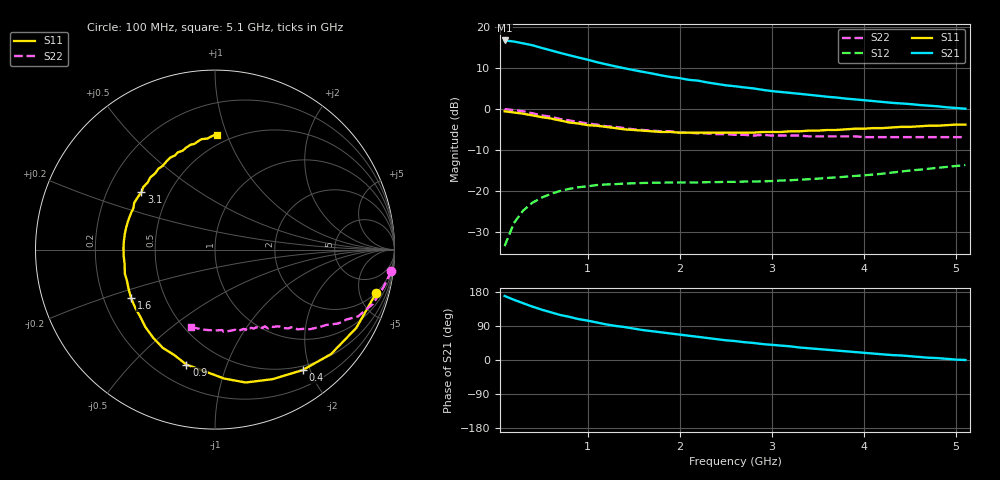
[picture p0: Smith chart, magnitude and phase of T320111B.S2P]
!AT-32011
!S PARAMETERSat Vce=1 V  Ic=2mA.  LAST UPDATED 01-05-95
# ghz s ma r 50
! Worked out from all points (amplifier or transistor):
!   51 points, 100 MHz to 5.1 GHz, reference 50 ohm
!   highest |S21| = 16.7 dB at 100 MHz (marker M1)
!   |S21| within 3 dB of that: start of sweep to 696.7 MHz
!   unconditionally stable (mu >= 1): 2.379 GHz to end of sweep
!   at 900 MHz: K = 0.39, MSG = 15.8 dB, |S12| = -19.2 dB
!   at 2.6 GHz: K = 1.08, MAG = 10.0 dB, |S12| = -17.9 dB
!   at 5.1 GHz: K = 1.06, MAG = 5.4 dB, |S12| = -13.8 dB
!   S11 on the Smith chart (normalised r, x): 100 MHz: 1.98, -7.05; 400 MHz: 0.44, -1.88; 900 MHz: 0.32, -0.73; 1.6 GHz: 0.32, -0.24; 3.1 GHz: 0.35, +0.31; 5.1 GHz: 0.43, +0.92
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0.1  0.93 -15.0  6.81 169.0  0.021 82.0  0.99 -7.0
0.2  0.9 -29.0  6.61 159.0  0.04 74.0  0.96 -13.0
0.3  0.87 -42.0  6.28 150.0  0.057 66.0  0.93 -19.0
0.4  0.83 -54.0  5.96 141.0  0.071 60.0  0.88 -25.0
0.5  0.79 -66.0  5.53 133.0  0.082 54.0  0.83 -28.0
0.6  0.76 -77.0  5.16 126.0  0.091 49.0  0.8 -31.0
0.7  0.72 -86.0  4.81 119.0  0.099 45.0  0.75 -34.0
0.9  0.66 -104.0  4.22 108.0  0.11 38.0  0.69 -40.0
1  0.63 -111.0  3.97 104.0  0.113 36.0  0.66 -42.0
1.2  0.6 -125.0  3.49 94.0  0.119 32.0  0.61 -45.0
1.3  0.58 -132.0  3.29 90.0  0.12 30.0  0.6 -47.0
1.6  0.54 -150.0  2.82 79.0  0.124 26.0  0.55 -51.0
1.8  0.52 -161.0  2.55 73.0  0.125 25.0  0.53 -54.0
2.1  0.51 -176.0  2.25 64.0  0.126 24.0  0.51 -59.0
2.2  0.51 179.0  2.2 61.0  0.126 24.0  0.5 -60.0
2.5  0.51 166.0  1.93 52.0  0.128 24.0  0.49 -64.0
2.6  0.51 162.0  1.88 50.0  0.128 24.0  0.48 -65.0
2.9  0.52 150.0  1.7 42.0  0.13 25.0  0.48 -69.0
3.1  0.52 142.0  1.6 38.0  0.133 26.0  0.47 -72.0
3.5  0.54 128.0  1.44 29.0  0.14 29.0  0.46 -78.0
4.3  0.59 106.0  1.18 13.0  0.166 33.0  0.45 -90.0
5.1  0.64 89.0  1 0.0  0.205 31.0  0.45 -107.0
